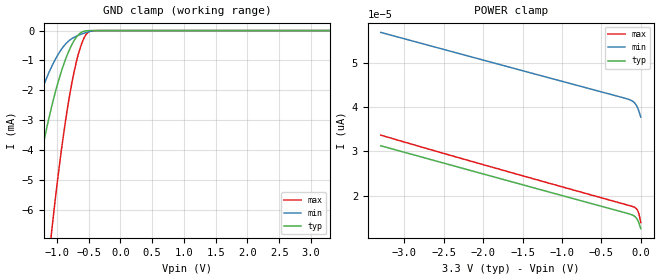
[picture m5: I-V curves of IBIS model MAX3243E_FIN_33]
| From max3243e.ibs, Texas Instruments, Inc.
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[Model]   MAX3243E_FIN_33
Model_type  Input
Vinl=0.8
Vinh=2.0
| variable   typ   min   max
C_comp   2.15pF   1.81pF   2.31pF
[Temperature Range]   40   100   -40
| Ambient temperature   25   85   -40
[Voltage range]   3.3   3   3.6
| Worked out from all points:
|   GND clamp passes 1 mA (typ) near -0.87 V on its own axis
[GND Clamp]
| MAX3243E_FIN_33
|   Voltage   I(typ)   I(min)   I(max)
-3.3V     -46.23mA   -28.95mA   -82.83mA
-1.81V    -12.1mA    -6.644mA   -25.91mA
-1.455V   -6.699mA   -3.471mA   -15.47mA
-1.27V    -4.436mA   -2.208mA   -10.82mA
-1.1V     -2.722mA   -1.297mA   -7.12mA
-1.07V    -2.458mA   -1.162mA   -6.53mA
-935mV    -1.42mA    -654.2uA   -4.134mA
-805mV    -663.7uA   -335.7uA   -2.265mA
-695mV    -231.9uA   -193.1uA   -1.081mA
-590mV    -35.84uA   -102.3uA   -339.1uA
-395mV    -43.53nA   -4.739uA   -796.1nA
3.3V      12.57pA    42.44pA    9.911pA
[POWER Clamp]
| MAX3243E_FIN_33
|   Voltage   I(typ)   I(min)   I(max)
-3.3V     31.25pA    56.79pA    33.65pA
-2.045V   25.12pA    50.77pA    27.22pA
-170mV    16.02pA    41.8pA     17.9pA
-125mV    15.77pA    41.5pA     17.67pA
-95mV     15.55pA    41.18pA    17.5pA
-70mV     15.24pA    40.74pA    17.29pA
-50mV     14.82pA    40.17pA    16.96pA
-35mV     14.33pA    39.59pA    16.47pA
-25mV     13.91pA    39.11pA    15.96pA
-15mV     13.41pA    38.58pA    15.26pA
-48.03fV  12.57pA    37.72pA    13.95pA
